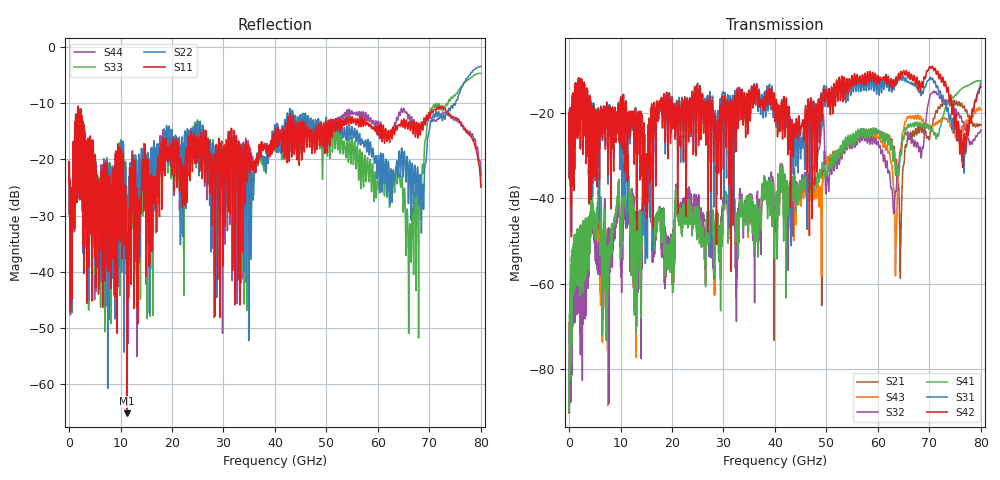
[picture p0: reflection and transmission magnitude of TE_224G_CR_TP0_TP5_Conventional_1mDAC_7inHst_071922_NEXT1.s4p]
!! Reference: tracy_3df_01a_2207
!! CHANNEL DESCRIPTION: TP0_TP5 CR Channel using 1meter DAC, Conventional 7in Host
!! MODEL DESCRIPTION: s4p, NEXT1
!! CONNECTOR DESCRIPTION: OSFP 200G SMT
!! CABLE DESCRIPTION: 1meter 26AWG Cable
!! MODEL STATUS: Developmental
!! PORT DEFINITIONS:
!! Port  1  ----->  Side A  Side B  <-----  Port  2
!! Port  3  ----->  Side A  Side B  <-----  Port  4
# GHz S MA R 50
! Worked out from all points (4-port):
!   8000 points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, 10 MHz to 80 GHz, reference 50 ohm
!   strongest paths, dB at 10 MHz, 20.01 GHz, 40.01 GHz, 60.01 GHz, 80 GHz:
!     S42: -26.6, -17.0, -22.1, -11.4, -13.9
!     S31: -26.6, -16.2, -17.4, -12.4, -12.9
!     S41: -84.4, -58.0, -43.5, -24.8, -12.6
!     S32: -87.5, -56.6, -45.9, -26.7, -24.0
!     S43: -86.1, -56.1, -42.9, -25.5, -19.3
!     S21: -86.1, -56.4, -44.1, -24.1, -22.8
!   lowest |S11| = -65.2 dB at 11.3 GHz (marker M1), VSWR 1.00, Z = 50 - j0.0496 ohm
!   |S11| at or under -10 dB: start of sweep to end of sweep
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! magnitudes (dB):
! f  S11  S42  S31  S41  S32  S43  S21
! 10 MHz  -24.3  -26.6  -26.6  -84.4  -87.5  -86.1  -86.1
! 4.41 GHz  -22.4  -21.4  -20.4  -35.8  -34.7  -35.0  -35.3
! 11.3 GHz  -65.2  -29.4  -29.0  -41.7  -44.1  -43.2  -43.3
! 59.4 GHz  -14.8  -11.1  -12.6  -24.9  -27.2  -25.9  -24.6
! 63.42 GHz  -14.0  -12.2  -12.3  -34.6  -38.2  -56.8  -32.0
! 66.19 GHz  -14.0  -11.7  -13.1  -22.9  -25.1  -20.7  -25.3
! 80 GHz  -24.9  -13.9  -12.9  -12.6  -24.0  -19.3  -22.8
